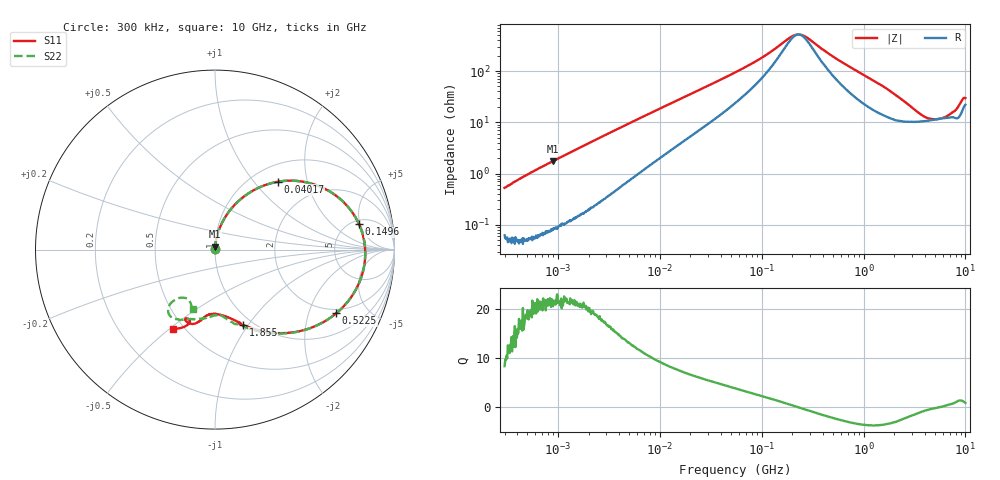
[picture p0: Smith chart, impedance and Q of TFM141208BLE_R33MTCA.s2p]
! S-Parameter Data Generated by TDK Corporation
! Copyright(C) 2026 TDK Corporation.
! All Rights Reserved.
! TDK P/N: TFM141208BLE-R33MTCA (SMD / SMT Inductor (Coil))
! Property: L=0.33uH at 1MHz
! Size(LxWxT): 1.4x1.2x0.8mm
! Model Type: s2p (Touchstone File Format Version 1.0)
! Frequency: DC=Yes Start=0.3MHz Stop=10000MHz 802points Log-sweep
! Model Generated on Feb. 24, 2026
! Terms and conditions regarding TDK Simulation Models:
! 1)This simulation model is being provided solely for informational
!  purposes. Please refer to the specifications of the products in
!  terms of detailed characteristics of such products.
! 2)In no event shall TDK Corporation of any of its subsidiaries be
!  liable for any loss or damage arising, directly or indirectly,
!  from any information contained in this simulation model, including,
!  but not limited to loss or damages arising from any inaccuracies,
!  omissions or errors in connection with such information.
! 3)Any and all copyrights on this simulation model are owned by
!  TDK Corporation.  Duplication or redistribution of this simulation
!  model without prior written permission from TDK Corporation
!  is prohibited.
! 4)This simulation model is subject to any modification or change
!  without any prior notice.
! 5)Neither TDK Corporation nor any of its subsidiaries shall make any
!  warranty, express or implied, including but not limited to the
!  correctness, implied warranties of merchantability and fitness for
!  a particular purpose with respect to this simulation models.
! 6)The use of this simulation model shall be deemed to have consented
!  to the terms and conditions hereof.
! Port Assignments:
!  1 ---@@@--- 2
! Applicable Conditions:
!  Temperature = 25 degC
!  DC Bias Current = 0 A
!  Small Signal Operation
# Hz S MA R 50
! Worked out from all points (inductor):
!   801 points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, 300 kHz to 10 GHz, reference 50 ohm
!   read as one part in series: L = 295 nH near 318.3 kHz
!   highest Q = 21.7 at 893.8 kHz (marker M1), where L = 310 nH
!   self-resonance near 230.3 MHz
!   S11 on the Smith chart (normalised r, x): 300 kHz: 1.00, +0.01; 40.17 MHz: 1.30, +1.34; 149.6 MHz: 5.71, +4.79; 522.5 MHz: 1.80, -3.07; 1.855 GHz: 0.90, -0.94; 10 GHz: 0.44, -0.52
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300000  0.003668 81.8  0.9993 -0.4  0.9995 -0.4  0.003725 78.0
567737  0.009965 86.5  0.9993 -0.7  0.9995 -0.7  0.009941 86.2
893778  0.01675 86.1  0.9989 -1.0  0.9991 -1.0  0.0167 86.1
1713600  0.03273 85.3  0.9977 -1.9  0.998 -1.9  0.03273 85.1
9671944  0.1718 73.9  0.9669 -9.9  0.967 -9.9  0.1718 73.9
1.968205e7  0.3137 63.1  0.9038 -18.3  0.904 -18.3  0.3136 63.1
4.016538e7  0.516 47.1  0.7549 -30.7  0.755 -30.7  0.516 47.1
5.477226e7  0.6086 38.7  0.6545 -36.7  0.6546 -36.7  0.6086 38.7
9.444554e7  0.7441 23.2  0.443 -44.5  0.443 -44.5  0.744 23.2
1.495617e8  0.8149 10.0  0.2599 -40.7  0.2599 -40.7  0.8149 10.0
2.22675e8  0.8373 -1.6  0.1631 -6.9  0.1631 -6.9  0.8376 -1.5
3.126428e8  0.8273 -11.7  0.2167 30.0  0.2168 30.0  0.8278 -11.6
5.225392e8  0.7629 -27.8  0.4101 39.1  0.4102 39.1  0.7642 -27.5
9.445544e8  0.6246 -47.8  0.6338 27.7  0.6339 27.7  0.6291 -47.5
1.767019e9  0.4593 -68.1  0.7896 9.5  0.7898 9.4  0.4647 -68.6
1.854885e9  0.4475 -69.7  0.7979 7.9  0.7981 7.9  0.4529 -70.1
2.924554e9  0.3734 -82.0  0.8385 -6.5  0.8387 -6.5  0.3729 -83.7
4.516006e9  0.3682 -97.0  0.8241 -21.1  0.8241 -21.1  0.3761 -94.3
7.316673e9  0.4312 -111.6  0.7676 -42.4  0.7681 -42.5  0.4385 -117.4
8.211115e9  0.4136 -112.3  0.7646 -48.2  0.7655 -48.3  0.4335 -127.0
9.105558e9  0.4261 -109.1  0.7598 -55.2  0.7594 -55.4  0.3373 -126.7
1e10  0.4989 -117.7  0.6754 -60.5  0.6755 -60.5  0.3555 -110.6
